| IBIS file was generated by Viper version: 2022.02.23
[IBIS Ver]   4.2
[Comment Char]   |_char
[File Name]   n9xx_n5xx_150mhz_184mapbga_9x9_p02g.ibs
[File Rev]   1.0
[Date]   Wed Feb 23 23:23:46 2022
[Source]   NXP Viper 2022.02.23
[Notes]
[Disclaimer] IMPORTANT NOTICE
  This information is provided on an AS IS basis and without warranty.
  IN NO EVENT SHALL NXP BE LIABLE FOR INCIDENTAL OR CONSEQUENTIAL
  DAMAGES ARISING FROM USE OF THIS INFORMATION. THIS DISCLAIMER OF
  WARRANTY EXTENDS TO THE USER OF THE INFORMATION, AND TO THEIR CUSTOMERS
  OR USERS OF PRODUCTS  AND IS IN LIEU OF ALL WARRANTIES WHETHER EXPRESS,
  IMPLIED, OR STATUTORY, INCLUDING IMPLIED WARRANTIES OF MERCHANTABILITY
  OR FITNESS FOR PARTICULAR PURPOSE.
  NXP does not represent or warrant that the information furnished
  hereunder is free of infringement of any third party patents,
  copyrights, trade secrets, or other intellectual property rights.
  NXP does not represent or warrant that the information is free of
  defect, or that it meets any particular standard, requirements or need
  of the user of the infomation or their customers.
  NXP reserves the right to change the information in this file
  without notice.
   http://www.nxp.com
[Copyright]   (C) Copyright NXP 2004 - 2022, All Rights Reserved.
|   n9xx_n5xx_150mhz_184mapbga_9x9_p02g
[Component]   n9xx_n5xx_150mhz_184mapbga_9x9_p02g
[Manufacturer]   NXP
[Package]
| variable   typ   min   max
R_pkg   0.12076   0.043974   0.22625
L_pkg   2.139e-09   1.092e-09   3.763e-09
C_pkg   4.411e-13   3.206e-13   7.916e-13
[Pin] signal_name   model_name   R_pin   L_pin   C_pin
A1   P1_8   a_ip_io_3v_3p3v   0.121   2.203e-09 4.080e-13
A2   P1_7   a_ip_io_3v_3p3v   0.13676   2.538e-09 3.999e-13
A4   P1_4   a_ip_io_3v_3p3v   0.14015   2.110e-09 3.868e-13
A6   P0_25   a_ip_io_3v_3p3v   0.11298   2.166e-09 3.826e-13
A8   P0_21   a_ip_io_3v_3p3v   0.093996  1.479e-09 3.378e-13
A10   P0_17   a_ip_io_3v_3p3v   0.12711   2.439e-09 3.556e-13
A12   P0_9   a_ip_io_3v_3p3v   0.10773   2.066e-09 3.474e-13
A14   P0_5   a_ip_io_3v_3p3v   0.11639   2.277e-09 3.856e-13
A16   P0_1   a_ip_io_3v_3p3v   0.14547   2.981e-09 4.352e-13
A17   P0_0   a_ip_io_3v_3p3v   0.15079   2.550e-09 4.415e-13
B1   P1_9   a_ip_io_3v_3p3v   0.12848   2.083e-09 3.941e-13
B2   P1_6   a_ip_io_3v_3p3v   0.13127   1.962e-09 4.007e-13
B3   P1_5   a_ip_io_3v_3p3v   0.11923   2.090e-09 3.958e-13
B4   P1_3   a_ip_io_3v_3p3v   0.11155   1.896e-09 3.772e-13
B6   P0_24   a_ip_io_3v_3p3v   0.11149   1.885e-09 3.567e-13
B7   P0_23   a_ip_io_3v_3p3v   0.11324   2.021e-09 3.499e-13
B8   P0_22   a_ip_io_3v_3p3v   0.085798  1.513e-09 3.349e-13
B10   P0_16   a_ip_io_3v_3p3v   0.10582   2.192e-09 3.624e-13
B11   P0_11   a_ip_io_3v_3p3v   0.088703  1.451e-09 3.706e-13
B12   P0_10   a_ip_io_3v_3p3v   0.097045  1.514e-09 3.704e-13
B14   P0_4   a_ip_io_3v_3p3v   0.13934   2.718e-09 4.207e-13
B15   P0_3   a_ip_io_3v_3p3v   0.1164   2.288e-09 4.058e-13
B16   P0_2   a_ip_io_3v_3p3v   0.13436   2.369e-09 4.025e-13
B17   P3_0   a_ip_io_3v_1p8v   0.12444   2.130e-09 4.101e-13
C3   P1_10   a_ip_io_3v_3p3v   0.09656   1.581e-09 3.943e-13
C4   P1_2   a_ip_io_3v_3p3v   0.12473   2.118e-09 4.134e-13
C5   P1_1   a_ip_io_3v_3p3v   0.09168   1.577e-09 3.774e-13
C6   P1_0   a_ip_io_3v_3p3v   0.15873   2.596e-09 4.254e-13
C8   P0_20   a_ip_io_3v_3p3v   0.068562  1.092e-09 3.640e-13
C9   P0_19   a_ip_io_3v_3p3v   0.085583  1.348e-09 3.206e-13
C10   P0_18   a_ip_io_3v_3p3v   0.088045  1.793e-09 3.328e-13
C12   P0_8   a_ip_io_3v_3p3v   0.10911   1.976e-09 3.806e-13
C13   P0_7   a_ip_io_3v_3p3v   0.10812   2.256e-09 4.191e-13
C14   P0_6   a_ip_io_3v_3p3v   0.1191   1.970e-09 4.270e-13
C15   P3_1   a_ip_io_3v_1p8v   0.10547   1.638e-09 4.323e-13
D1   P1_13   a_ip_io_3v_3p3v   0.13234   2.300e-09 4.039e-13
D2   P1_12   a_ip_io_3v_3p3v   0.11918   2.323e-09 4.153e-13
D3   P1_11   a_ip_io_3v_3p3v   0.12193   2.024e-09 4.049e-13
D4   P1_14   a_ip_io_3v_3p3v   0.087504  1.398e-09 4.480e-13
D6   VSS   GND   NA   NA   NA
D7   P0_31   a_ip_io_3v_3p3v   0.094943  1.711e-09 5.470e-13
D9   VSS   GND   NA   NA   NA
D11   P0_12   a_ip_io_3v_3p3v   0.1207   1.865e-09 5.852e-13
D12   VSS   GND   NA   NA   NA
D14   P3_7   a_ip_io_3v_1p8v   0.11422   1.929e-09 4.836e-13
D15   P3_2   a_ip_io_3v_1p8v   0.11021   1.684e-09 4.064e-13
D16   P3_3   a_ip_io_3v_1p8v   0.10482   1.839e-09 3.805e-13
D17   P3_6   a_ip_io_3v_1p8v   0.1226   1.951e-09 3.859e-13
E4   P1_15   a_ip_io_3v_3p3v   0.1118   1.718e-09 3.867e-13
E5   VSS   GND   NA   NA   NA
E7   P0_30   a_ip_io_3v_3p3v   0.13897   2.589e-09 5.718e-13
E8   P0_28   a_ip_io_3v_3p3v   0.14645   2.835e-09 6.209e-13
E10   P0_27   a_ip_io_3v_3p3v   0.1225   2.736e-09 6.292e-13
E11   P0_14   a_ip_io_3v_3p3v   0.10628   1.850e-09 5.674e-13
E13   VSS   GND   NA   NA   NA
E14   P3_8   a_ip_io_3v_1p8v   0.12584   2.019e-09 4.951e-13
F1   P1_30   a_ip_io_3v_3p3v   0.12641   2.323e-09 4.016e-13
F2   P1_31   a_ip_io_3v_3p3v   0.123   1.997e-09 3.856e-13
F3   RESET_B   a_ip_io_3v_3p3v   0.14959   2.845e-09 4.919e-13
F4   P1_17   a_ip_io_3v_3p3v   0.1137   2.009e-09 4.362e-13
F6   P1_16   a_ip_io_3v_3p3v   0.09467   1.424e-09 5.519e-13
F8   P0_29   a_ip_io_3v_3p3v   0.11056   2.021e-09 5.838e-13
F10   P0_26   a_ip_io_3v_3p3v   0.17131   3.296e-09 6.648e-13
F12   P0_13   a_ip_io_3v_3p3v   0.14824   2.752e-09 5.396e-13
F14   P3_4   a_ip_io_3v_1p8v   0.11498   1.953e-09 4.221e-13
F15   P3_9   a_ip_io_3v_1p8v   0.11914   2.382e-09 4.157e-13
F16   P3_11   a_ip_io_3v_1p8v   0.094292  1.612e-09 3.710e-13
F17   P3_10   a_ip_io_3v_1p8v   0.12799   2.238e-09 3.847e-13
G2   VSS   GND   NA   NA   NA
G4   P1_18   a_ip_io_3v_3p3v   0.10596   1.698e-09 4.722e-13
G5   P1_19   a_ip_io_3v_3p3v   0.12909   2.353e-09 5.358e-13
G7   VDD   POWER   NA   NA   NA
G11   VDD_P3   POWER   NA   NA   NA
G13   P0_15   a_ip_io_3v_3p3v   0.1745   3.568e-09 6.146e-13
G14   P3_5   a_ip_io_3v_1p8v   0.12173   2.285e-09 4.404e-13
G16   P3_12   a_ip_io_3v_1p8v   0.11035   1.750e-09 3.611e-13
H1   P2_1   a_ip_io_3v_1p8v   0.13016   2.317e-09 3.933e-13
H2   P2_0   a_ip_io_3v_1p8v   0.1162   1.790e-09 3.880e-13
H3   P2_2   a_ip_io_3v_1p8v   0.13629   2.699e-09 4.136e-13
H5   VSS   GND   NA   NA   NA
H6   VDD   POWER   NA   NA   NA
H8   VDD   POWER   NA   NA   NA
H9   VSS   GND   NA   NA   NA
H10   VDD_P3   POWER   NA   NA   NA
H12   VDD_P3   POWER   NA   NA   NA
H13   VSS   GND   NA   NA   NA
H15   P3_15   a_ip_io_3v_1p8v   0.11309   2.107e-09 3.968e-13
H16   P3_13   a_ip_io_3v_1p8v   0.079448  1.255e-09 3.575e-13
H17   P3_14   a_ip_io_3v_1p8v   0.12283   2.169e-09 3.494e-13
J3   P2_3   a_ip_io_3v_1p8v   0.10601   2.100e-09 3.806e-13
J4   VSS   GND   NA   NA   NA
J8   VSS   GND   NA   NA   NA
J10   VSS   GND   NA   NA   NA
J14   VSS   GND   NA   NA   NA
J15   P3_16   a_ip_io_3v_1p8v   0.10223   1.642e-09 3.718e-13
K1   P2_5   a_ip_io_3v_1p8v   0.13509   2.373e-09 3.843e-13
K2   P2_6   a_ip_io_3v_1p8v   0.11384   1.784e-09 3.703e-13
K3   P2_4   a_ip_io_3v_1p8v   0.079326  1.244e-09 3.827e-13
K5   P1_20   a_ip_io_3v_3p3v   0.1833   3.763e-09 6.887e-13
K6   VDD_LDO_CORE   POWER   NA   NA   NA
K8   VDD_P2   POWER   NA   NA   NA
K9   VSS   GND   NA   NA   NA
K10   VDD_CORE   POWER   NA   NA   NA
K12   P5_5   a_ip_io_3v_1p8v   0.22625   3.669e-09 7.916e-13
K13   P5_6   a_ip_io_3v_1p8v   0.21183   3.525e-09 7.297e-13
K15   P3_17   a_ip_io_3v_1p8v   0.1152   2.178e-09 4.298e-13
K16   P3_18   NC   0.13484   2.422e-09 4.016e-13
K17   P3_19   a_ip_io_3v_1p8v   0.12827   2.065e-09 3.948e-13
L2   P2_7   a_ip_io_3v_1p8v   0.10217   1.830e-09 3.706e-13
L4   P1_22   a_ip_io_3v_3p3v   0.17144   3.375e-09 6.892e-13
L5   P1_21   a_ip_io_3v_3p3v   0.15037   3.046e-09 7.600e-13
L7   VDD_P2   POWER   NA   NA   NA
L11   VDD_CORE   POWER   NA   NA   NA
L13   P5_7   a_ip_io_3v_1p8v   0.17869   3.165e-09 6.352e-13
L14   P5_8   a_ip_io_3v_1p8v   0.18106   3.235e-09 6.345e-13
L16   P3_21   a_ip_io_3v_1p8v   0.1067   1.692e-09 3.353e-13
M1   P2_9   a_ip_io_3v_1p8v   0.10484   1.899e-09 3.563e-13
M2   P2_8   a_ip_io_3v_1p8v   0.10915   1.749e-09 3.689e-13
M3   P2_10   a_ip_io_3v_1p8v   0.11762   1.820e-09 4.078e-13
M4   P1_23   a_ip_io_3v_3p3v   0.15799   3.255e-09 4.953e-13
M6   P4_4   a_ip_io_3v_3p3v   0.1583   2.707e-09 6.289e-13
M8   P4_5   a_ip_io_3v_3p3v   0.15706   3.056e-09 6.156e-13
M10   P5_2   a_ip_io_3v_1p8v   0.16105   2.802e-09 6.347e-13
M12   P5_4   a_ip_io_3v_1p8v   0.14971   2.272e-09 7.527e-13
M14   P5_9   a_ip_io_3v_1p8v   0.1569   2.605e-09 5.746e-13
M15   P3_23   a_ip_io_3v_1p8v   0.11432   1.896e-09 5.062e-13
M16   P3_22   a_ip_io_3v_1p8v   0.10593   2.049e-09 3.507e-13
M17   P3_20   a_ip_io_3v_1p8v   0.1274   2.528e-09 3.703e-13
N4   P2_11   a_ip_io_3v_1p8v   0.10379   1.599e-09 4.455e-13
N5   VDD_P4   POWER   NA   NA   NA
N7   P4_6   a_ip_io_3v_3p3v   0.11971   2.268e-09 4.778e-13
N8   P4_14   a_ip_io_3v_3p3v   0.098105  1.709e-09 4.879e-13
N10   P4_18   a_ip_io_3v_3p3v   0.10946   2.085e-09 4.673e-13
N11   P5_3   a_ip_io_3v_1p8v   0.16235   2.652e-09 7.013e-13
N13   VSS   GND   NA   NA   NA
N14   VDD_SYS   POWER   NA   NA   NA
P1   P4_0   a_ip_io_3v_3p3v   0.1331   2.206e-09 3.882e-13
P2   P4_1   a_ip_io_3v_3p3v   0.14044   2.583e-09 4.274e-13
P3   ANA_0   NC   0.098406  1.690e-09 3.907e-13
P4   VDD_P4   POWER   NA   NA   NA
P6   VSS_P4   GND   NA   NA   NA
P7   VSS_P4   GND   NA   NA   NA
P9   VSS_P4   GND   NA   NA   NA
P11   USB1_ID   NC   0.072494  1.238e-09 4.656e-13
P12   VSS   GND   NA   NA   NA
P14   VSS   GND   NA   NA   NA
P15   VDD_LDO_SYS   POWER   NA   NA   NA
P16   VSS_DCDC   GND   NA   NA   NA
P17   DCDC_LX   NC   0.043974  1.235e-09 4.766e-13
R3   ANA_1   NC   0.10232   1.710e-09 4.146e-13
R4   VDD_ANA   POWER   NA   NA   NA
R5   VREFH   POWER   0.056588  1.349e-09 4.652e-13
R6   VREFL   GND   0.12017   1.809e-09 3.699e-13
R8   P4_16   a_ip_io_3v_3p3v   0.0671   1.109e-09 3.539e-13
R9   P4_17   a_ip_io_3v_3p3v   0.10046   1.639e-09 3.854e-13
R10   P4_19   a_ip_io_3v_3p3v   0.070265  1.266e-09 3.857e-13
R12   VDD_USB   POWER   NA   NA   NA
R13   USB1_DP   NC   0.15159   2.961e-09 4.558e-13
R14   USB1_DM   NC   0.15002   3.113e-09 4.846e-13
R15   VDD_DCDC   POWER   NA   NA   NA
T1   P4_2   a_ip_io_3v_3p3v   0.13976   2.791e-09 4.226e-13
T2   ANA_4   NC   0.12439   1.949e-09 4.039e-13
T3   ANA_5   NC   0.1219   1.922e-09 4.088e-13
T4   P4_7   a_ip_io_3v_3p3v   0.10823   1.608e-09 3.576e-13
T6   P4_12   a_ip_io_3v_3p3v   0.10309   1.533e-09 3.547e-13
T7   P4_13   a_ip_io_3v_3p3v   0.09692   1.580e-09 3.688e-13
T8   P4_15   a_ip_io_3v_3p3v   0.095429  1.497e-09 3.545e-13
T10   P4_20   a_ip_io_3v_3p3v   0.084617  1.222e-09 3.427e-13
T11   P4_21   a_ip_io_3v_3p3v   0.092081  1.690e-09 3.555e-13
T12   P4_22   a_ip_io_3v_3p3v   0.10263   2.025e-09 3.830e-13
T14   USB0_DM   NC   0.13084   2.233e-09 3.972e-13
T15   USB0_DP   NC   0.13867   2.252e-09 4.154e-13
T16   VSS   GND   NA   NA   NA
T17   VDD_BAT   POWER   NA   NA   NA
U1   P4_3   a_ip_io_3v_3p3v   0.12697   2.320e-09 3.946e-13
U2   ANA_6   NC   0.13242   2.446e-09 4.027e-13
U4   ANA_7   NC   0.072895  1.854e-09 3.384e-13
U6   ANA_14   NC   0.11531   1.993e-09 3.753e-13
U8   ANA_18   NC   0.094232  1.817e-09 3.570e-13
U10   ANA_22   NC   0.12134   2.198e-09 3.668e-13
U12   P4_23   a_ip_io_3v_3p3v   0.12562   2.191e-09 3.921e-13
U14   USB1_VBUS   POWER   0.12942   2.451e-09 4.578e-13
U16   P5_0   a_ip_io_3v_1p8v   0.1728   3.052e-09 4.694e-13
U17   P5_1   a_ip_io_3v_1p8v   0.16325   2.864e-09 4.806e-13
[Pin Mapping]   pulldown_ref   pullup_ref
A1   NC   NC
A2   NC   NC
A4   NC   NC
A6   NC   NC
A8   NC   NC
A10   NC   NC
A12   NC   NC
A14   NC   NC
A16   NC   NC
A17   NC   NC
B1   NC   NC
B2   NC   NC
B3   NC   NC
B4   NC   NC
B6   NC   NC
B7   NC   NC
B8   NC   NC
B10   NC   NC
B11   NC   NC
B12   NC   NC
B14   NC   NC
B15   NC   NC
B16   NC   NC
B17   NC   NC
C3   NC   NC
C4   NC   NC
C5   NC   NC
C6   NC   NC
C8   NC   NC
C9   NC   NC
C10   NC   NC
C12   NC   NC
C13   NC   NC
C14   NC   NC
C15   NC   NC
D1   NC   NC
D2   NC   NC
D3   NC   NC
D4   NC   NC
D6   VSS   NC
D7   NC   NC
D9   VSS   NC
D11   NC   NC
D12   VSS   NC
D14   NC   NC
D15   NC   NC
D16   NC   NC
D17   NC   NC
E4   NC   NC
E5   VSS   NC
E7   NC   NC
E8   NC   NC
E10   NC   NC
E11   NC   NC
E13   VSS   NC
E14   NC   NC
F1   NC   NC
F2   NC   NC
F3   NC   NC
F4   NC   NC
F6   NC   NC
F8   NC   NC
F10   NC   NC
F12   NC   NC
F14   NC   NC
F15   NC   NC
F16   NC   NC
F17   NC   NC
G2   VSS   NC
G4   NC   NC
G5   NC   NC
G7   NC   VDD
G11   NC   VDD_P3
G13   NC   NC
G14   NC   NC
G16   NC   NC
H1   NC   NC
H2   NC   NC
H3   NC   NC
H5   VSS   NC
H6   NC   VDD
H8   NC   VDD
H9   VSS   NC
H10   NC   VDD_P3
H12   NC   VDD_P3
H13   VSS   NC
H15   NC   NC
H16   NC   NC
H17   NC   NC
J3   NC   NC
J4   VSS   NC
J8   VSS   NC
J10   VSS   NC
J14   VSS   NC
J15   NC   NC
K1   NC   NC
K2   NC   NC
K3   NC   NC
K5   NC   NC
K6   NC   VDD_LDO_CORE
K8   NC   VDD_P2
K9   VSS   NC
K10   NC   VDD_CORE
K12   NC   NC
K13   NC   NC
K15   NC   NC
K16   NC   NC
K17   NC   NC
L2   NC   NC
L4   NC   NC
L5   NC   NC
L7   NC   VDD_P2
L11   NC   VDD_CORE
L13   NC   NC
L14   NC   NC
L16   NC   NC
M1   NC   NC
M2   NC   NC
M3   NC   NC
M4   NC   NC
M6   NC   NC
M8   NC   NC
M10   NC   NC
M12   NC   NC
M14   NC   NC
M15   NC   NC
M16   NC   NC
M17   NC   NC
N4   NC   NC
N5   NC   VDD_P4
N7   NC   NC
N8   NC   NC
N10   NC   NC
N11   NC   NC
N13   VSS   NC
N14   NC   VDD_SYS
P1   NC   NC
P2   NC   NC
P3   NC   NC
P4   NC   VDD_P4
P6   VSS_P4   NC
P7   VSS_P4   NC
P9   VSS_P4   NC
P11   NC   NC
P12   VSS   NC
P14   VSS   NC
P15   NC   VDD_LDO_SYS
P16   VSS_DCDC   NC
P17   NC   NC
R3   NC   NC
R4   NC   VDD_ANA
R5   NC   VREFH
R6   VREFL   NC
R8   NC   NC
R9   NC   NC
R10   NC   NC
R12   NC   VDD_USB
R13   NC   NC
R14   NC   NC
R15   NC   VDD_DCDC
T1   NC   NC
T2   NC   NC
T3   NC   NC
T4   NC   NC
T6   NC   NC
T7   NC   NC
T8   NC   NC
T10   NC   NC
T11   NC   NC
T12   NC   NC
T14   NC   NC
T15   NC   NC
T16   VSS   NC
T17   NC   VDD_BAT
U1   NC   NC
U2   NC   NC
U4   NC   NC
U6   NC   NC
U8   NC   NC
U10   NC   NC
U12   NC   NC
U14   NC   USB1_VBUS
U16   NC   NC
U17   NC   NC
|*   Model Selector   *
[Model Selector] a_ip_io_3v_1p8v
p_io_25mhz_ds0_sr0_1p8v_mio   dse=0 sre=0 25mhz
p_io_25mhz_ds0_sr1_1p8v_mio   dse=0 sre=1 25mhz
p_io_25mhz_ds1_sr0_1p8v_mio   dse=1 sre=0 25mhz
p_io_25mhz_ds1_sr1_1p8v_mio   dse=1 sre=1 25mhz
p_io_25mhz_r40_ds0_sr0_1p8v_mio   dse=0 sre=0 25mhz_r40
p_io_25mhz_r40_ds0_sr1_1p8v_mio   dse=0 sre=1 25mhz_r40
p_io_25mhz_r40_ds1_sr0_1p8v_mio   dse=1 sre=0 25mhz_r40
p_io_25mhz_r40_ds1_sr1_1p8v_mio   dse=1 sre=1 25mhz_r40
p_io_50mhz_ds0_sr0_1p8v_mio   dse=0 sre=0 50mhz
p_io_50mhz_ds0_sr1_1p8v_mio   dse=0 sre=1 50mhz
p_io_50mhz_ds1_sr0_1p8v_mio   dse=1 sre=0 50mhz
p_io_50mhz_ds1_sr1_1p8v_mio   dse=1 sre=1 50mhz
p_io_25mhz_cap_ds0_sr0_1p8v_mio   dse=0 sre=0 25mhz_cap
p_io_25mhz_cap_ds0_sr1_1p8v_mio   dse=0 sre=1 25mhz_cap
p_io_25mhz_cap_ds1_sr0_1p8v_mio   dse=1 sre=0 25mhz_cap
p_io_25mhz_cap_ds1_sr1_1p8v_mio   dse=1 sre=1 25mhz_cap
p_io_25mhz_2mux_ds0_sr0_1p8v_mio   dse=0 sre=0 25mhz_2mux
p_io_25mhz_2mux_ds0_sr1_1p8v_mio   dse=0 sre=1 25mhz_2mux
p_io_25mhz_2mux_ds1_sr0_1p8v_mio   dse=1 sre=0 25mhz_2mux
p_io_25mhz_2mux_ds1_sr1_1p8v_mio   dse=1 sre=1 25mhz_2mux
p_io_100mhz_ds0_sr0_1p8v_mio   dse=0 sre=0 100mhz
p_io_100mhz_ds0_sr1_1p8v_mio   dse=0 sre=1 100mhz
p_io_100mhz_ds1_sr0_1p8v_mio   dse=1 sre=0 100mhz
p_io_100mhz_ds1_sr1_1p8v_mio   dse=1 sre=1 100mhz
p_io_100mhz_weftd_ds0_sr0_1p8v_mio   dse=0 sre=0 100mhz
p_io_100mhz_weftd_ds0_sr1_1p8v_mio   dse=0 sre=1 100mhz
p_io_100mhz_weftd_ds1_sr0_1p8v_mio   dse=1 sre=0 100mhz
p_io_100mhz_weftd_ds1_sr1_1p8v_mio   dse=1 sre=1 100mhz
p_io_i2c_ds00_ds10_sr0_1p8v_mio   dse0=0 dse1=0 sre=0 i2c
p_io_i2c_ds00_ds10_sr1_1p8v_mio   dse0=0 dse1=0 sre=1 i2c
p_io_i2c_ds00_ds11_sr0_1p8v_mio   dse0=0 dse1=1 sre=0 i2c
p_io_i2c_ds00_ds11_sr1_1p8v_mio   dse0=0 dse1=1 sre=1 i2c
p_io_i2c_ds01_ds10_sr0_1p8v_mio   dse0=1 dse1=0 sre=0 i2c
p_io_i2c_ds01_ds10_sr1_1p8v_mio   dse0=1 dse1=0 sre=1 i2c
p_io_i2c_ds01_ds11_sr0_1p8v_mio   dse0=1 dse1=1 sre=0 i2c
p_io_i2c_ds01_ds11_sr1_1p8v_mio   dse0=1 dse1=1 sre=1 i2c
p_io_i2c_i2c1_1p8v_mio   ipp_i2c_lv=1 i2c
p_io_i2cfmp_ds00_ds10_sr0_1p8v_mio   dse0=0 dse1=0 sre=0 i2cfmp
p_io_i2cfmp_ds00_ds10_sr1_1p8v_mio   dse0=0 dse1=0 sre=1 i2cfmp
p_io_i2cfmp_ds00_ds11_sr0_1p8v_mio   dse0=0 dse1=1 sre=0 i2cfmp
p_io_i2cfmp_ds00_ds11_sr1_1p8v_mio   dse0=0 dse1=1 sre=1 i2cfmp
p_io_i2cfmp_ds01_ds10_sr0_1p8v_mio   dse0=1 dse1=0 sre=0 i2cfmp
p_io_i2cfmp_ds01_ds10_sr1_1p8v_mio   dse0=1 dse1=0 sre=1 i2cfmp
p_io_i2cfmp_ds01_ds11_sr0_1p8v_mio   dse0=1 dse1=1 sre=0 i2cfmp
p_io_i2cfmp_ds01_ds11_sr1_1p8v_mio   dse0=1 dse1=1 sre=1 i2cfmp
p_io_i2cfmp_i2c1_1p8v_mio   ipp_i2c_lv=1 i2cfmp
p_io_rst_1p8v_mio   rst
p_io_rst_rx1p8v_1p8v_mio   rst
p_io_aon_1p8v_mio   rst
[Model Selector] a_ip_io_3v_3p3v
p_io_25mhz_ds0_sr0_3p3v_mio   dse=0 sre=0 25mhz
p_io_25mhz_ds0_sr1_3p3v_mio   dse=0 sre=1 25mhz
p_io_25mhz_ds1_sr0_3p3v_mio   dse=1 sre=0 25mhz
p_io_25mhz_ds1_sr1_3p3v_mio   dse=1 sre=1 25mhz
p_io_25mhz_r40_ds0_sr0_3p3v_mio   dse=0 sre=0 25mhz_r40
p_io_25mhz_r40_ds0_sr1_3p3v_mio   dse=0 sre=1 25mhz_r40
p_io_25mhz_r40_ds1_sr0_3p3v_mio   dse=1 sre=0 25mhz_r40
p_io_25mhz_r40_ds1_sr1_3p3v_mio   dse=1 sre=1 25mhz_r40
p_io_50mhz_ds0_sr0_3p3v_mio   dse=0 sre=0 50mhz
p_io_50mhz_ds0_sr1_3p3v_mio   dse=0 sre=1 50mhz
p_io_50mhz_ds1_sr0_3p3v_mio   dse=1 sre=0 50mhz
p_io_50mhz_ds1_sr1_3p3v_mio   dse=1 sre=1 50mhz
p_io_25mhz_cap_ds0_sr0_3p3v_mio   dse=0 sre=0 25mhz_cap
p_io_25mhz_cap_ds0_sr1_3p3v_mio   dse=0 sre=1 25mhz_cap
p_io_25mhz_cap_ds1_sr0_3p3v_mio   dse=1 sre=0 25mhz_cap
p_io_25mhz_cap_ds1_sr1_3p3v_mio   dse=1 sre=1 25mhz_cap
p_io_25mhz_2mux_ds0_sr0_3p3v_mio   dse=0 sre=0 25mhz_2mux
p_io_25mhz_2mux_ds0_sr1_3p3v_mio   dse=0 sre=1 25mhz_2mux
p_io_25mhz_2mux_ds1_sr0_3p3v_mio   dse=1 sre=0 25mhz_2mux
p_io_25mhz_2mux_ds1_sr1_3p3v_mio   dse=1 sre=1 25mhz_2mux
p_io_100mhz_ds0_sr0_3p3v_mio   dse=0 sre=0 100mhz
p_io_100mhz_ds0_sr1_3p3v_mio   dse=0 sre=1 100mhz
p_io_100mhz_ds1_sr0_3p3v_mio   dse=1 sre=0 100mhz
p_io_100mhz_ds1_sr1_3p3v_mio   dse=1 sre=1 100mhz
p_io_100mhz_weftd_ds0_sr0_3p3v_mio   dse=0 sre=0 100mhz
p_io_100mhz_weftd_ds0_sr1_3p3v_mio   dse=0 sre=1 100mhz
p_io_100mhz_weftd_ds1_sr0_3p3v_mio   dse=1 sre=0 100mhz
p_io_100mhz_weftd_ds1_sr1_3p3v_mio   dse=1 sre=1 100mhz
p_io_i2c_ds00_ds10_sr0_3p3v_mio   dse0=0 dse1=0 sre=0 i2c
p_io_i2c_ds00_ds10_sr1_3p3v_mio   dse0=0 dse1=0 sre=1 i2c
p_io_i2c_ds00_ds11_sr0_3p3v_mio   dse0=0 dse1=1 sre=0 i2c
p_io_i2c_ds00_ds11_sr1_3p3v_mio   dse0=0 dse1=1 sre=1 i2c
p_io_i2c_ds01_ds10_sr0_3p3v_mio   dse0=1 dse1=0 sre=0 i2c
p_io_i2c_ds01_ds10_sr1_3p3v_mio   dse0=1 dse1=0 sre=1 i2c
p_io_i2c_ds01_ds11_sr0_3p3v_mio   dse0=1 dse1=1 sre=0 i2c
p_io_i2c_ds01_ds11_sr1_3p3v_mio   dse0=1 dse1=1 sre=1 i2c
p_io_i2c_i2c1_3p3v_mio   ipp_i2c_lv=1 i2c
p_io_i2cfmp_ds00_ds10_sr0_3p3v_mio   dse0=0 dse1=0 sre=0 i2cfmp
p_io_i2cfmp_ds00_ds10_sr1_3p3v_mio   dse0=0 dse1=0 sre=1 i2cfmp
p_io_i2cfmp_ds00_ds11_sr0_3p3v_mio   dse0=0 dse1=1 sre=0 i2cfmp
p_io_i2cfmp_ds00_ds11_sr1_3p3v_mio   dse0=0 dse1=1 sre=1 i2cfmp
p_io_i2cfmp_ds01_ds10_sr0_3p3v_mio   dse0=1 dse1=0 sre=0 i2cfmp
p_io_i2cfmp_ds01_ds10_sr1_3p3v_mio   dse0=1 dse1=0 sre=1 i2cfmp
p_io_i2cfmp_ds01_ds11_sr0_3p3v_mio   dse0=1 dse1=1 sre=0 i2cfmp
p_io_i2cfmp_ds01_ds11_sr1_3p3v_mio   dse0=1 dse1=1 sre=1 i2cfmp
p_io_i2cfmp_i2c1_3p3v_mio   ipp_i2c_lv=1 i2cfmp
p_io_rst_3p3v_mio   rst
p_io_rst_rx1p8v_3p3v_mio   rst
p_io_aon_3p3v_mio   rst
| End [Component] n9xx_n5xx_150mhz_184mapbga_9x9_p02g
| Models and submodels in the file (98): p_io_100mhz_ds0_sr0_1p8v_mio (I/O), p_io_100mhz_ds0_sr0_3p3v_mio (I/O), p_io_100mhz_ds0_sr1_1p8v_mio (I/O), p_io_100mhz_ds0_sr1_3p3v_mio (I/O), p_io_100mhz_ds1_sr0_1p8v_mio (I/O), p_io_100mhz_ds1_sr0_3p3v_mio (I/O), p_io_100mhz_ds1_sr1_1p8v_mio (I/O), p_io_100mhz_ds1_sr1_3p3v_mio (I/O), p_io_100mhz_weftd_ds0_sr0_1p8v_mio (I/O), p_io_100mhz_weftd_ds0_sr0_3p3v_mio (I/O), p_io_100mhz_weftd_ds0_sr1_1p8v_mio (I/O), p_io_100mhz_weftd_ds0_sr1_3p3v_mio (I/O), p_io_100mhz_weftd_ds1_sr0_1p8v_mio (I/O), p_io_100mhz_weftd_ds1_sr0_3p3v_mio (I/O), p_io_100mhz_weftd_ds1_sr1_1p8v_mio (I/O), p_io_100mhz_weftd_ds1_sr1_3p3v_mio (I/O), p_io_25mhz_2mux_ds0_sr0_1p8v_mio (I/O), p_io_25mhz_2mux_ds0_sr0_3p3v_mio (I/O), p_io_25mhz_2mux_ds0_sr1_1p8v_mio (I/O), p_io_25mhz_2mux_ds0_sr1_3p3v_mio (I/O), p_io_25mhz_2mux_ds1_sr0_1p8v_mio (I/O), p_io_25mhz_2mux_ds1_sr0_3p3v_mio (I/O), p_io_25mhz_2mux_ds1_sr1_1p8v_mio (I/O), p_io_25mhz_2mux_ds1_sr1_3p3v_mio (I/O), p_io_25mhz_cap_ds0_sr0_1p8v_mio (I/O), p_io_25mhz_cap_ds0_sr0_3p3v_mio (I/O), p_io_25mhz_cap_ds0_sr1_1p8v_mio (I/O), p_io_25mhz_cap_ds0_sr1_3p3v_mio (I/O), p_io_25mhz_cap_ds1_sr0_1p8v_mio (I/O), p_io_25mhz_cap_ds1_sr0_3p3v_mio (I/O), p_io_25mhz_cap_ds1_sr1_1p8v_mio (I/O), p_io_25mhz_cap_ds1_sr1_3p3v_mio (I/O), p_io_25mhz_ds0_sr0_1p8v_mio (I/O), p_io_25mhz_ds0_sr0_3p3v_mio (I/O), p_io_25mhz_ds0_sr1_1p8v_mio (I/O), p_io_25mhz_ds0_sr1_3p3v_mio (I/O), p_io_25mhz_ds1_sr0_1p8v_mio (I/O), p_io_25mhz_ds1_sr0_3p3v_mio (I/O), p_io_25mhz_ds1_sr1_1p8v_mio (I/O), p_io_25mhz_ds1_sr1_3p3v_mio (I/O), p_io_25mhz_r40_ds0_sr0_1p8v_mio (I/O), p_io_25mhz_r40_ds0_sr0_3p3v_mio (I/O), p_io_25mhz_r40_ds0_sr1_1p8v_mio (I/O), p_io_25mhz_r40_ds0_sr1_3p3v_mio (I/O), p_io_25mhz_r40_ds1_sr0_1p8v_mio (I/O), p_io_25mhz_r40_ds1_sr0_3p3v_mio (I/O), p_io_25mhz_r40_ds1_sr1_1p8v_mio (I/O), p_io_25mhz_r40_ds1_sr1_3p3v_mio (I/O), p_io_50mhz_ds0_sr0_1p8v_mio (I/O), p_io_50mhz_ds0_sr0_3p3v_mio (I/O), p_io_50mhz_ds0_sr1_1p8v_mio (I/O), p_io_50mhz_ds0_sr1_3p3v_mio (I/O), p_io_50mhz_ds1_sr0_1p8v_mio (I/O), p_io_50mhz_ds1_sr0_3p3v_mio (I/O), p_io_50mhz_ds1_sr1_1p8v_mio (I/O), p_io_50mhz_ds1_sr1_3p3v_mio (I/O), p_io_aon_1p8v_mio (I/O), p_io_aon_3p3v_mio (I/O), p_io_i2c_ds00_ds10_sr0_1p8v_mio (I/O), p_io_i2c_ds00_ds10_sr0_3p3v_mio (I/O), p_io_i2c_ds00_ds10_sr1_1p8v_mio (I/O), p_io_i2c_ds00_ds10_sr1_3p3v_mio (I/O), p_io_i2c_ds00_ds11_sr0_1p8v_mio (I/O), p_io_i2c_ds00_ds11_sr0_3p3v_mio (I/O), p_io_i2c_ds00_ds11_sr1_1p8v_mio (I/O), p_io_i2c_ds00_ds11_sr1_3p3v_mio (I/O), p_io_i2c_ds01_ds10_sr0_1p8v_mio (I/O), p_io_i2c_ds01_ds10_sr0_3p3v_mio (I/O), p_io_i2c_ds01_ds10_sr1_1p8v_mio (I/O), p_io_i2c_ds01_ds10_sr1_3p3v_mio (I/O), p_io_i2c_ds01_ds11_sr0_1p8v_mio (I/O), p_io_i2c_ds01_ds11_sr0_3p3v_mio (I/O), p_io_i2c_ds01_ds11_sr1_1p8v_mio (I/O), p_io_i2c_ds01_ds11_sr1_3p3v_mio (I/O), p_io_i2c_i2c1_1p8v_mio (I/O), p_io_i2c_i2c1_3p3v_mio (I/O), p_io_i2cfmp_ds00_ds10_sr0_1p8v_mio (I/O), p_io_i2cfmp_ds00_ds10_sr0_3p3v_mio (I/O), p_io_i2cfmp_ds00_ds10_sr1_1p8v_mio (I/O), p_io_i2cfmp_ds00_ds10_sr1_3p3v_mio (I/O)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
